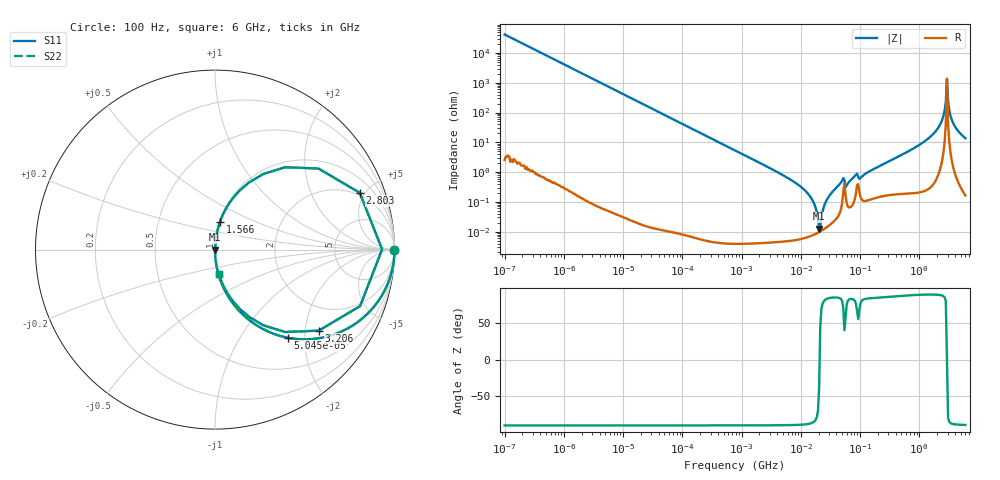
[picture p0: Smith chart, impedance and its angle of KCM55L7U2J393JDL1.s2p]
!Murata Part Number: KCM55L7U2J393JDL1
!These Parameters are Measured in Series Mode Connection
!Data Generated on Mar 13, 2026
!  o--ll--o
!Port1  Port2
!  o------o
!Operation Temp=25[degC], DC Bias Voltage=0[V]
!Freq. Start=100[Hz] Stop=6[GHz] 401[Steps]
# Hz S RI R 50
!Freq.(Hz) S11(Real) S11(Imag) S21(Real) S21(Imag) S12(Real) S12(Imag) S22(Real) S22(Imag)
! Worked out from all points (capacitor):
!   401 points, 100 Hz to 6 GHz, reference 50 ohm
!   read as one part in series: C = 38.2 nF near 109 Hz
!   lowest |Z| = 12.7 mohm at 20.35 MHz (marker M1)
!   series resonance near 20.77 MHz, so ESL is about 1.5 nH
!   S11 on the Smith chart (normalised r, x): 100 Hz: open; 50.45 kHz: 1.00, -1.65; 1.566 GHz: 1.01, +0.32; 2.803 GHz: 1.81, +4.61; 3.206 GHz: 1.21, -2.37; 6 GHz: 1.00, -0.28
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100  1 -0.0024  5.9e-06 0.0024  5.9e-06 0.0024  1 -0.0024
2008  0.9977 -0.0481  0.00232 0.0481  0.00232 0.0481  0.9977 -0.0481
13169  0.9093 -0.2871  0.0907 0.2871  0.0907 0.2871  0.9093 -0.2871
40335  0.5167 -0.4997  0.4833 0.4997  0.4833 0.4997  0.5167 -0.4997
50455  0.4059 -0.491  0.5941 0.491  0.5941 0.491  0.4059 -0.491
141303  0.0802 -0.2715  0.9198 0.2715  0.9198 0.2715  0.0802 -0.2715
774597  0.00292 -0.0536  0.9971 0.0536  0.9971 0.0536  0.00292 -0.0536
7266822  7.55e-05 -0.00504  0.9999 0.00504  0.9999 0.00504  7.55e-05 -0.00504
1.555665e7  7.61e-05 -0.00118  0.9999 0.00118  0.9999 0.00118  7.61e-05 -0.00118
2.035112e7  9.68e-05 -8.15e-05  0.9999 8.15e-05  0.9999 8.15e-05  9.68e-05 -8.15e-05
2.911731e7  0.000156 0.00141  0.9998 -0.00141  0.9998 -0.00141  0.000156 0.00141
4.983056e7  0.000921 0.00507  0.9991 -0.00507  0.9991 -0.00507  0.000921 0.00507
6.233367e7  0.000714 0.00411  0.9993 -0.00411  0.9993 -0.00411  0.000714 0.00411
3.124326e8  0.00221 0.023  0.9978 -0.023  0.9978 -0.023  0.00221 0.023
1.565993e9  0.0275 0.1538  0.9725 -0.1538  0.9725 -0.1538  0.0275 0.1538
2.240541e9  0.1404 0.332  0.8596 -0.332  0.8596 -0.332  0.1404 0.332
2.562649e9  0.3901 0.4588  0.6099 -0.4588  0.6099 -0.4588  0.3901 0.4588
2.802721e9  0.8069 0.3162  0.1931 -0.3162  0.1931 -0.3162  0.8069 0.3162
3.205649e9  0.5784 -0.4514  0.4216 0.4514  0.4216 0.4514  0.5784 -0.4514
3.352442e9  0.3919 -0.4593  0.6081 0.4593  0.6081 0.4593  0.3919 -0.4593
3.8344e9  0.1413 -0.3335  0.8587 0.3335  0.8587 0.3335  0.1413 -0.3335
6e9  0.0201 -0.1345  0.9799 0.1345  0.9799 0.1345  0.0201 -0.1345
